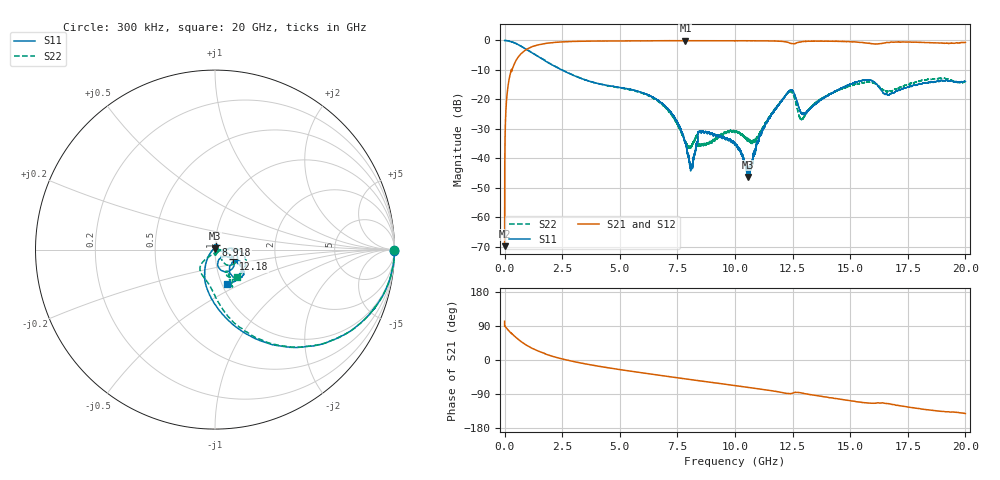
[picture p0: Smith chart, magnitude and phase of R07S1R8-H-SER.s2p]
!{R07S1R8}
!Johanson Technology Inc.
!www.johansontechnology.com
!Test Board Conditions:
!Substrate Type  RO4350B
!Substrate Thickness  10 mil
!Substrate Dk  3.66
!TL Type: GCPW
!TL Trace Width  21 mil
!TL Gap  20 mil
!Electrode orientation  Horizontal
!DUT TOPOLOGY	SERIES
!Mounting Pad LxW  16x21 mil
! Created Sat Feb  6 11:23:00 2021
# hz S ma R 50
! 2 Port Network Data from SP1.SP block
! freq  magS11  angS11  magS21  angS21  magS12  angS12  magS22  angS22
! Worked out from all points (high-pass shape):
!   20001 points, 300 kHz to 20 GHz, reference 50 ohm
!   highest |S21| = -0.06 dB at 7.85 GHz (marker M1); lowest = -69.8 dB at 300 kHz (marker M2)
!   |S21| within 3 dB of the highest: 946.2 MHz to end of sweep
!   lowest |S11| = -46.3 dB at 10.57 GHz (marker M3), VSWR 1.01, Z = 50.1 + j0.476 ohm
!   |S11| at or under -10 dB: 2.481 GHz to end of sweep
!   |S22| runs from -36.6 to 0.0 dB; largest |S21 - S12| = 0.011
!   S11 on the Smith chart (normalised r, x): 300 kHz: open; 8.918 GHz: 1.01, +0.05; 12.18 GHz: 1.22, -0.13; 20 GHz: 1.05, -0.42
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300000  0.9974 -0.4  0.0003224 102.3  0.0003605 83.5  0.9969 -0.2
1.013e8  0.9919 -7.3  0.1155 82.9  0.1156 82.9  0.992 -7.2
1.313e8  0.9881 -9.5  0.1492 80.6  0.1491 80.8  0.9883 -9.5
4.883e8  0.8878 -29.9  0.4507 59.9  0.4506 59.7  0.8898 -29.7
1.7123e9  0.4657 -73.0  0.8793 17.8  0.8784 17.7  0.4716 -70.8
3.3343e9  0.2258 -100.9  0.9696 -8.2  0.9691 -8.3  0.2269 -94.0
6.6673e9  0.0958 -123.0  0.9883 -39.8  0.9884 -39.8  0.09247 -134.6
7.4113e9  0.04673 -136.6  0.9901 -46.1  0.991 -46.1  0.04337 -127.5
7.8503e9  0.0183 -158.4  0.9929 -49.8  0.991 -49.8  0.01868 -96.7
8.1103e9  0.006489 128.1  0.9912 -52.0  0.9914 -52.0  0.01582 -39.7
8.4873e9  0.02773 57.8  0.9902 -55.1  0.9904 -55.1  0.01638 5.5
8.9183e9  0.02651 76.0  0.9888 -58.6  0.9889 -58.6  0.01929 -37.1
1.00003e10  0.01778 117.8  0.988 -67.5  0.9897 -67.5  0.02816 -89.4
1.05673e10  0.004834 79.3  0.9895 -72.1  0.9892 -72.1  0.02003 -73.3
1.12713e10  0.03348 -9.0  0.9847 -78.3  0.9855 -78.2  0.0352 -4.3
1.21773e10  0.1138 -26.7  0.9489 -87.4  0.9488 -87.3  0.1142 -7.3
1.24843e10  0.1422 -58.9  0.8844 -87.7  0.8816 -87.7  0.13 -39.5
1.28813e10  0.05805 -65.4  0.9472 -86.9  0.9496 -86.9  0.0456 -26.6
1.33343e10  0.07325 -31.2  0.9714 -91.9  0.9726 -92.0  0.07608 4.4
1.55743e10  0.2109 -41.1  0.9186 -112.7  0.919 -112.6  0.1906 -31.2
1.66673e10  0.1187 -37.2  0.92 -115.2  0.9229 -115.6  0.1384 -62.7
2e10  0.2023 -71.6  0.9283 -141.2  0.9233 -141.2  0.1955 -51.1
